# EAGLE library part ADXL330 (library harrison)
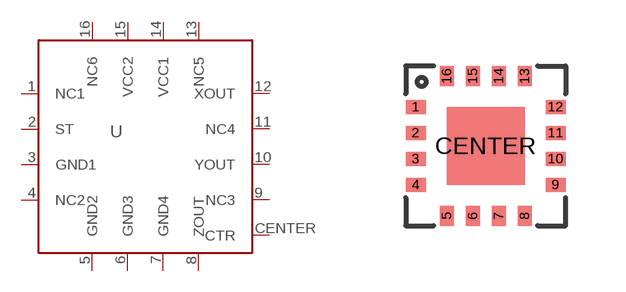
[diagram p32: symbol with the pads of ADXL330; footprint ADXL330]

Designator prefix U

## ADXL330  [ADXL330]
1  NC1
2  ST
3  GND1
4  NC2
5  GND2
6  GND3
7  GND4
8  ZOUT
9  NC3
10  YOUT
11  NC4
12  XOUT
13  NC5
14  VCC1
15  VCC2
16  NC6
CENTER  CTR

## Footprint ADXL330 (pad centres in mm)
smd 0.5 x 0.35: 1 -1.75,0.975; 2 -1.75,0.325; 3 -1.75,-0.325; 4 -1.75,-0.975; 9 1.75,-0.975; 10 1.75,-0.325; 11 1.75,0.325; 12 1.75,0.975
smd 0.35 x 0.5: 5 -0.975,-1.75; 6 -0.325,-1.75; 7 0.325,-1.75; 8 0.975,-1.75; 13 0.975,1.75; 14 0.325,1.75; 15 -0.325,1.75; 16 -0.975,1.75
smd 1.95 x 1.95: CENTER 0,0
